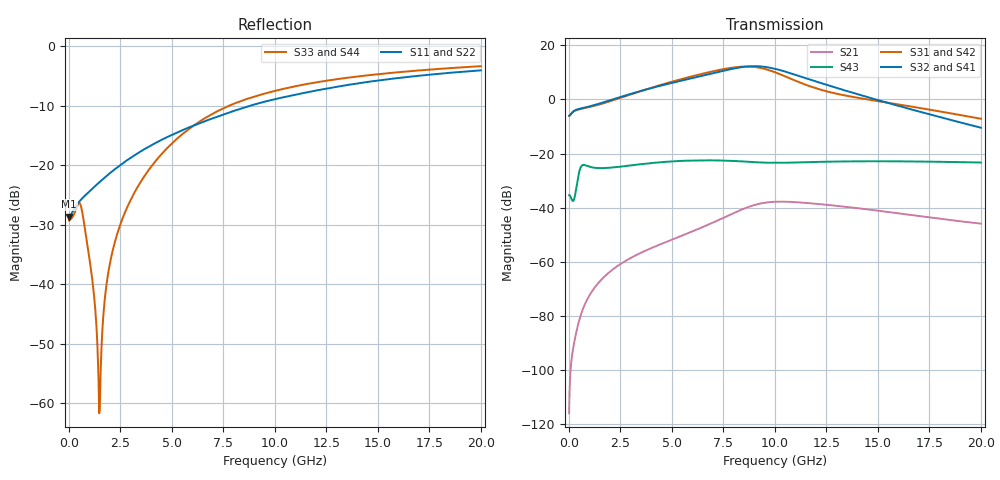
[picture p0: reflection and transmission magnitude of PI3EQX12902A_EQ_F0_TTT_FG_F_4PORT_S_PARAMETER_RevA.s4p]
! NPort=4 DATA=2000 NOISE=0 GROUPDELAY=0 COMPLEX_DATAFORMAT=POLAR
! NumOfBlock=1 NumOfParam=0
! .MODEL Smodel S TSTONEFILE=PI3EQX12902A_EQ_F0_TTT_FG_F_4PORT_S_PARAMETER_RevA.s4p TYPE=S
!  -- The above .MODEL line can be used for the S element in the netlist.
! The s parameter is extracted from the linear redriver, it is not bi-directional; only s(4,1)s(4,2) and s(3,1)s(3,2)
! should be the insertion loss
!Port definition:
!Port1 = input+
!Port2 = input-
!Port3 = output+
!Port4 = output-
# Hz S MA R  50
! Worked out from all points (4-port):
!   2000 points, 10 MHz to 20 GHz, reference 50 ohm
!   strongest paths, dB at 10 MHz, 5.01 GHz, 10.01 GHz, 15.01 GHz, 20 GHz:
!     S32: -6.0, 6.1, 11.3, -0.3, -10.4
!     S41: -6.0, 6.1, 11.2, -0.3, -10.4
!     S31: -6.0, 6.6, 10.0, -0.6, -7.1
!     S42: -6.0, 6.5, 9.8, -0.8, -7.2
!     S43: -35.3, -22.9, -23.4, -22.8, -23.3
!     S21: -116.0, -51.8, -37.8, -41.1, -45.9
!   lowest |S11| = -28.6 dB at 10 MHz (marker M1), VSWR 1.08, Z = 46.4 - j0.0607 ohm
!   |S11| at or under -10 dB: start of sweep to 8.807 GHz
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1e7  0.03704 -179.0  1.589e-06 51.9  0 0.0  0 0.0
     1.589e-06 51.9  0.03704 -179.0  0 0.0  0 0.0
     0.4992 1.0  0.4992 -179.0  0.03429 6.0  0.01709 -177.1
     0.4992 -179.0  0.4992 1.0  0.01709 -177.1  0.03429 6.0
6.01e9  0.2139 -112.0  0.003667 95.3  1.688e-06 -23.4  1.033e-06 87.1
        0.003665 95.2  0.2139 -112.0  1.036e-06 87.3  1.68e-06 -23.1
        2.696 -48.8  2.492 110.1  0.2125 -46.5  0.07407 144.6
        2.485 110.1  2.659 -49.4  0.07448 144.7  0.2119 -46.5
7.89e9  0.2816 -111.7  0.007631 78.1  6.728e-06 -79.8  4.235e-06 44.1
        0.007617 78.1  0.2815 -111.7  4.245e-06 44.1  6.696e-06 -79.4
        3.852 -101.6  3.647 57.3  0.3224 -65.1  0.07288 124.7
        3.627 57.2  3.788 -102.0  0.07336 124.6  0.3217 -65.0
9.24e9  0.3325 -113.3  0.01184 48.0  1.232e-05 -127.5  9.835e-06 -4.8
        0.01181 48.0  0.3325 -113.3  9.828e-06 -4.9  1.227e-05 -126.9
        3.864 -152.9  4.094 4.4  0.3881 -76.1  0.06822 114.5
        4.058 4.5  3.792 -153.3  0.06863 114.2  0.3877 -76.0
1.068e10  0.3812 -115.7  0.01289 11.9  1.553e-05 -166.7  1.502e-05 -61.5
          0.01285 12.0  0.3812 -115.7  1.495e-05 -61.6  1.555e-05 -165.8
          2.495 161.1  3.119 -50.5  0.4485 -85.4  0.06771 107.6
          3.085 -50.2  2.44 160.8  0.06796 107.3  0.4485 -85.3
1.307e10  0.4577 -119.5  0.01076 -26.8  2.289e-05 153.8  1.886e-05 -131.4
          0.01075 -26.4  0.4578 -119.5  1.871e-05 -131.2  2.309e-05 154.4
          1.259 126.6  1.601 -112.3  0.5297 -97.8  0.07137 92.0
          1.587 -111.6  1.227 126.9  0.07134 91.7  0.5301 -97.7
2e10  0.6263 -131.6  0.005024 -74.6  4.154e-05 50.7  1.803e-05 99.5
      0.005079 -74.7  0.6263 -131.6  1.783e-05 100.4  4.201e-05 50.8
      0.4399 39.7  0.3005 132.4  0.6794 -119.6  0.06845 46.2
      0.3017 133.3  0.435 40.4  0.06835 46.1  0.6797 -119.6
